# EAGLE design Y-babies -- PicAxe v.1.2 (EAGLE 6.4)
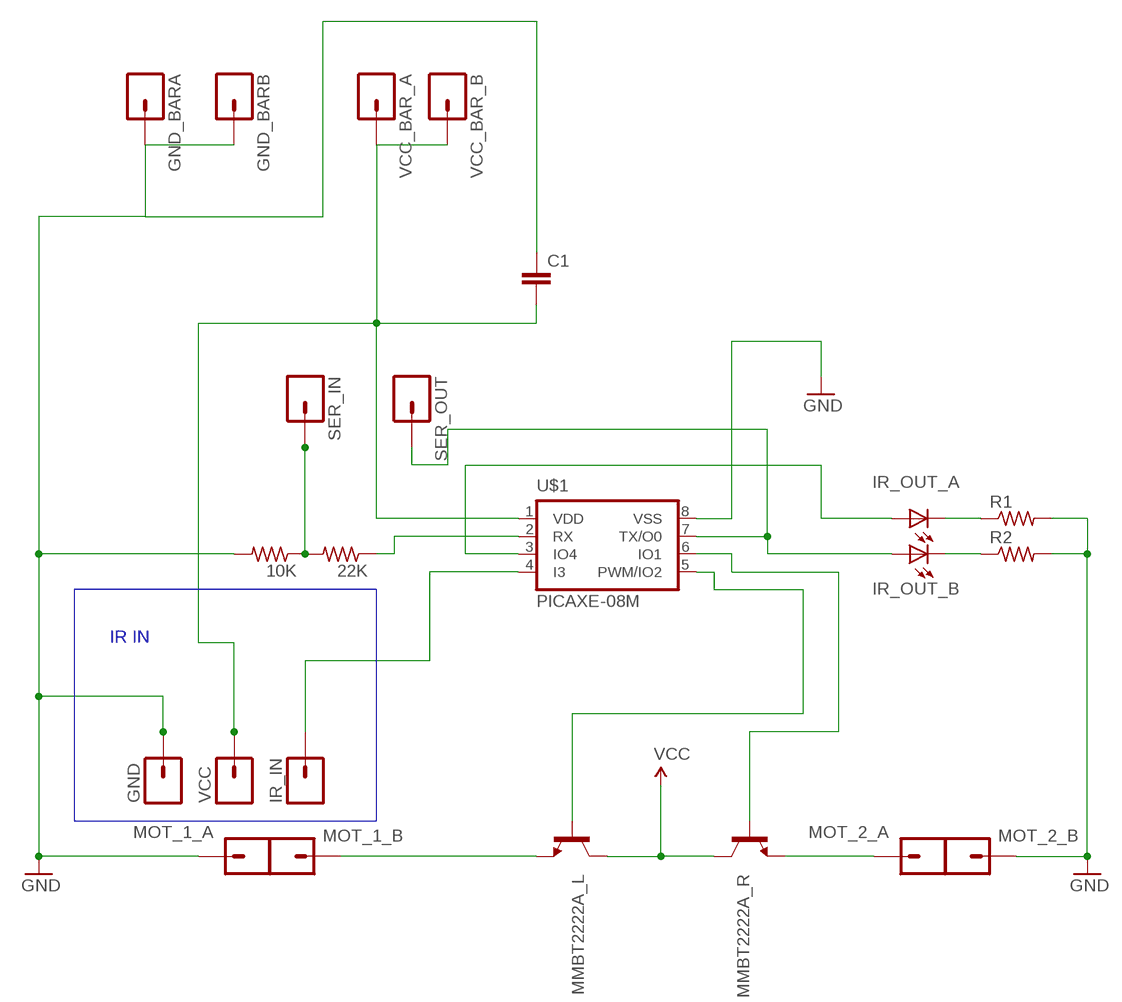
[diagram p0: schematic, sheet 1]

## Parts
10K  R-US_R0805W  [R0805W]
22K  R-US_R0805W  [R0805W]
C1  CAPPTH1  [CAP-PTH-5MM]
GND  M01PTH  [1X01]
GND_BARA  M01PTH  [1X01]
GND_BARB  M01PTH  [1X01]
IR_IN  M01PTH  [1X01]
IR_OUT_A  LED3MM  [LED3MM]
IR_OUT_B  LED3MM  [LED3MM]
MMBT2222A_L  TRANSISTOR_NPNSOT23  [SOT23]
MMBT2222A_R  TRANSISTOR_NPNSOT23  [SOT23]
MOT_1_A  M01SMD-4.5X1.5  [PAD-1.5X4.5]
MOT_1_B  M01SMD-4.5X1.5  [PAD-1.5X4.5]
MOT_2_A  M01SMD-4.5X1.5  [PAD-1.5X4.5]
MOT_2_B  M01SMD-4.5X1.5  [PAD-1.5X4.5]
R1  R-US_R0805W  [R0805W]
R2  R-US_R0805W  [R0805W]
SER_IN  M01PTH  [1X01]
SER_OUT  M01PTH  [1X01]
U$1  PICAXE-08M  [DIL8]
VCC  M01PTH  [1X01]
VCC_BAR_A  M01PTH  [1X01]
VCC_BAR_B  M01PTH  [1X01]

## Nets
GND: 10K.2 C1.1 GND.1 GND_BARA.1 GND_BARB.1 MOT_1_A.P$1 MOT_2_B.P$1 R1.2 R2.2 U$1.8(VSS)
N$1: MMBT2222A_L.1(B) U$1.5(PWM/IO2)
N$2: MMBT2222A_R.1(B) U$1.6(IO1)
N$3: IR_OUT_B.A SER_OUT.1 U$1.7(TX/O0)
N$4: IR_OUT_B.K(C) R2.1
N$5: 10K.1 22K.2 SER_IN.1
N$6: IR_OUT_A.A U$1.3(IO4)
N$7: IR_OUT_A.K(C) R1.1
N$8: 22K.1 U$1.2(RX)
N$9: MMBT2222A_L.2(E) MOT_1_B.P$1
N$10: MMBT2222A_R.2(E) MOT_2_A.P$1
N$11: IR_IN.1 U$1.4(I3)
VCC: C1.2 MMBT2222A_L.3(C) MMBT2222A_R.3(C) U$1.1(VDD) VCC.1 VCC_BAR_A.1 VCC_BAR_B.1

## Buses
B$1

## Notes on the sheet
- IR IN

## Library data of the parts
10K 22K R1 R2 = resistor:R-US_: RESISTOR, American symbol
C1 = SparkFun:CAP: Capacitor
GND GND_BARA GND_BARB IR_IN MOT_1_A MOT_1_B MOT_2_A MOT_2_B SER_IN SER_OUT VCC VCC_BAR_A VCC_BAR_B = SparkFun:M01: Header 1
IR_OUT_A IR_OUT_B = led:LED: LED
MMBT2222A_L MMBT2222A_R = SparkFun:TRANSISTOR_NPN: Transistor NPN BJT configuration in SOT23 package. MMBT2222 is the common NPN we use. Double check BCE configuration again layout.
U$1 = picaxe-3:PICAXE-08M

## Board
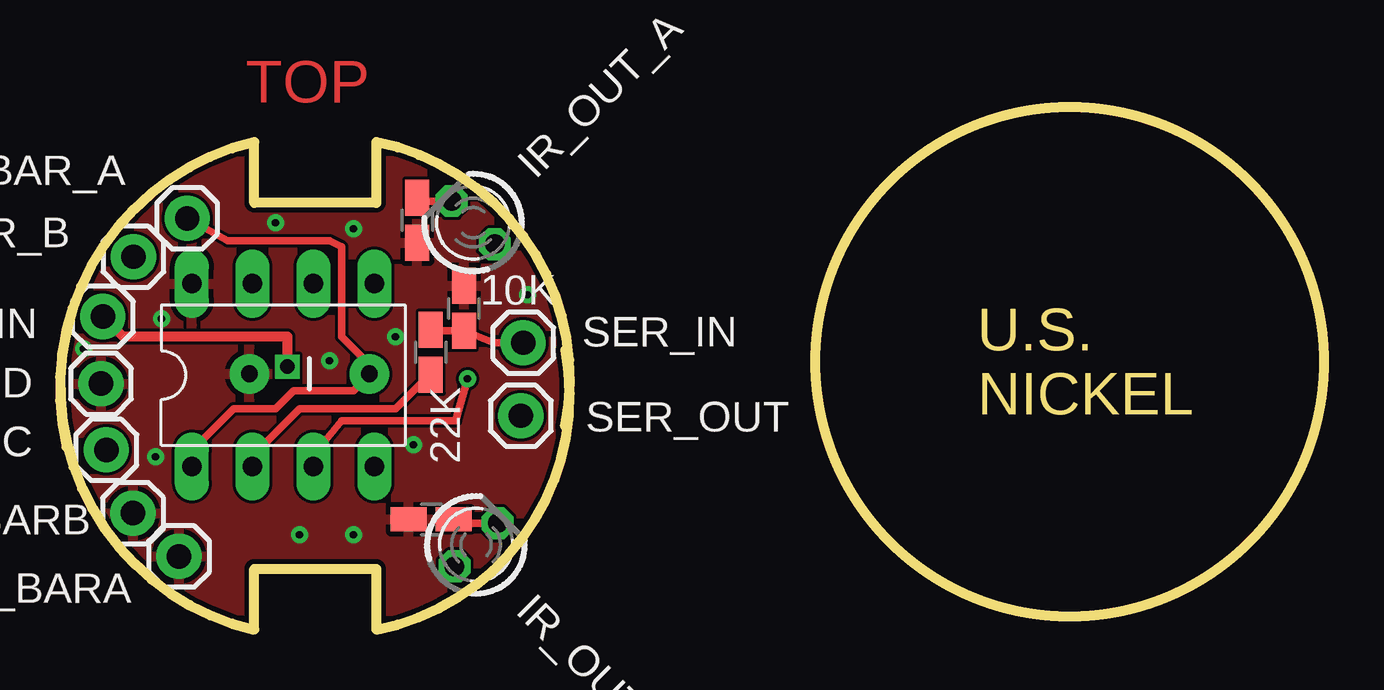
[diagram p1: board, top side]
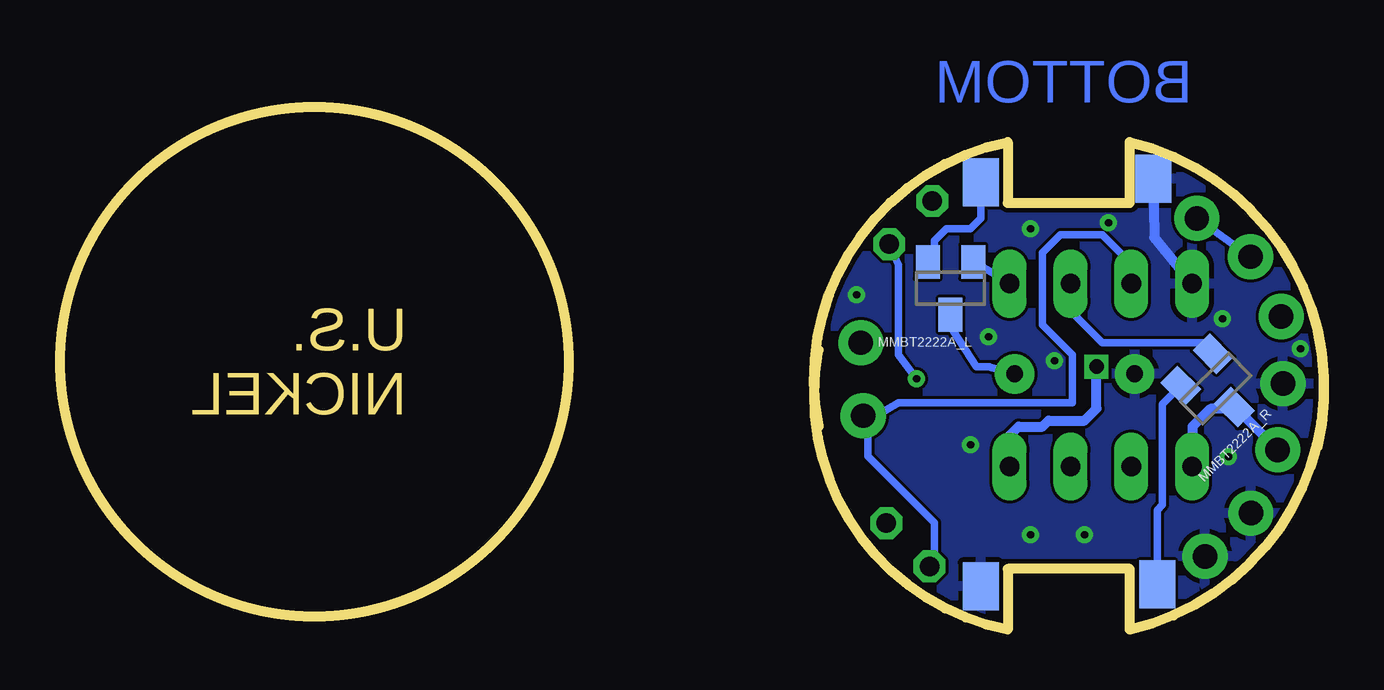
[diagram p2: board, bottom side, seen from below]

Size 52.69 x 21.77 mm. Coordinates in mm from the lower left corner, seen from the top.
Outline: 0.27,7.62 arc-90 8.1,20.32 8.1,17.78 13.18,17.78 13.18,20.32 arc-90 21.06,8.46
Outline: 0.27,12.48 arc90 8.1,0 8.1,2.54 13.18,2.54 13.18,0 arc90 21.07,11.66
Outline: circle at 42.08,11.16 radius 10.61
Copper layers (1*16): Top 0.035mm / dielectric 1.5mm / Bottom 0.035mm
Design rules "default *": minimum track width 10mil, minimum drill 24mil, track to track 5mil, track to pad 5mil, pad to pad 5mil, via to via 5mil, smd to smd 5mil, copper to edge 8mil, drill to drill 6mil, minimum pad ring 10mil, minimum via ring 8mil, stop-mask expansion 4mil, vias tented up to drill 0.3mm, thermal gap 8mil

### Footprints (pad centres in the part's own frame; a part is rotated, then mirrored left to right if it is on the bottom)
R0805W = smd 1.5 x 1: 1 -0.94,0; 2 0.94,0
CAP-PTH-5MM = drill 0.7 pad 1.651: 1 -2.5,0; 2 2.5,0
1X01 = drill 1.016 pad 1.88: 1 0,0
LED3MM = drill 0.813 octagon: A -1.27,0; K 1.27,0
SOT23 = smd 1 x 1.4: 1 -0.95,-1.1; 2 0.95,-1.1; 3 0,1.1
PAD-1.5X4.5 = smd 1.5 x 2: P$1 0,0
DIL8 = drill 0.813 pad 1.422 long: 1 -3.81,-3.81; 2 -1.27,-3.81; 3 1.27,-3.81; 4 3.81,-3.81; 5 3.81,3.81; 6 1.27,3.81; 7 -1.27,3.81; 8 -3.81,3.81

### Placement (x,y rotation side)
10K  16.84,13.39 90 top
22K  15.46,11.56 90 top
C1  10.39,10.66 0 top
GND  1.71,10.26 0 top
GND_BARA  4.96,3.05 0 top
GND_BARB  3.04,4.86 0 top
IR_IN  1.79,13.05 0 top
IR_OUT_A  17.22,16.96 135 top
IR_OUT_B  17.34,3.54 45 top
MMBT2222A_L  15.57,14.22 180 bottom
MMBT2222A_R  4.51,10.05 225 bottom
MOT_1_A  7.12,18.78 0 bottom
MOT_1_B  14.29,18.65 180 bottom
MOT_2_A  6.96,1.89 180 bottom
MOT_2_B  14.31,1.81 0 bottom
R1  14.89,17.06 270 top
R2  15.48,4.6 180 top
SER_IN  19.31,11.96 0 top
SER_OUT  19.21,8.92 0 top
U$1  9.3,10.61 0 top
VCC  1.93,7.49 0 top
VCC_BAR_A  5.3,17.14 0 top
VCC_BAR_B  3.06,15.54 0 top

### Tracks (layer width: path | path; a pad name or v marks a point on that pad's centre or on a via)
GND  (via drill 0.3)
  Bottom 0.406: MOT_1_A.P$1 7.08,16.35 U$1.8
  other vias: 9.98,3.96 0.98,11.71 14.73,7.71 12.23,16.71 19.48,13.96 4.23,12.96 13.98,12.21 11.23,11.21 8.98,16.96 12.23,3.96 3.98,7.21
  pour Bottom: -0.79,20.32 -0.79,0 22.07,0 22.07,20.32
  pour Top: -0.79,20.32 -0.79,0 22.07,0 22.07,20.32
N$1
  Bottom 0.305: MMBT2222A_L.1 13.71,14.81 U$1.5
N$2
  Bottom 0.305: U$1.6 10.57,13.3 9.23,11.96 5.08,11.96 MMBT2222A_R.1
N$3
  Bottom 0.305: U$1.7 8.03,15.26 9.23,16.46 10.98,16.46 11.73,15.71 11.73,12.71 10.48,11.46 10.48,9.46 17.73,9.46 19,8.71 | 19,8.71 SER_OUT.1 | 19,8.71 19,7.23 16.23,4.46 16.23,2.85 IR_OUT_B.A
N$4
  Top 0.305: IR_OUT_B.K 16.58,4.44 R2.1
N$5
  Top 0.305: SER_IN.1 18.08,11.95 10K.1 15.51,12.45 22K.2
N$6  (via drill 0.3)
  Top 0.305: U$1.3 10.57,7.3 11.73,8.71 16.48,8.71 v16.98,10.46
  Bottom 0.305: v16.98,10.46 17.73,11.46 17.73,15.2 IR_OUT_A.A
N$7
  Top 0.305: IR_OUT_A.K 15.03,17.86 R1.1
N$8
  Top 0.305: U$1.2 8.03,7.26 9.98,9.21 13.98,9.21 15.23,10.46 15.3,10.46 22K.1
N$9
  Bottom 0.305: MOT_1_B.P$1 14.29,17.15 14.73,16.71 15.73,16.71 16.23,16.21 16.23,15.61 MMBT2222A_L.2
N$10
  Bottom 0.305: MOT_2_A.P$1 6.96,4.99 6.73,5.21 6.73,9.39 MMBT2222A_R.2
N$11  (via drill 0.6)
  Top 0.406: v9.48,10.96 9.48,12.21 2.63,12.21 IR_IN.1
  Bottom 0.406: U$1.4 13.11,8.08 12.73,8.46 11.73,8.46 11.48,8.71 9.98,8.71 9.48,9.21 v9.48,10.96
VCC
  Top 0.305: 12.98,10.71 12.98,10.96 11.73,12.21 11.73,15.96 11.23,16.21 6.98,16.21 VCC_BAR_A.1 | 5.48,7.46 7.23,9.21 8.98,9.21 9.73,9.96 12.23,9.96 12.98,10.71 | 12.98,10.71 12.94,10.71 C1.2
  Top 0.406: U$1.1 5.49,7.45 5.48,7.46
  Bottom 0.305: MMBT2222A_L.3 15.45,12.43 14.48,10.96 13.98,10.96 | 13.98,10.96 13.94,10.96 | C1.2 12.93,10.66 13.98,10.96 | VCC_BAR_A.1 VCC_BAR_B.1 2.73,14.84 | MMBT2222A_R.3 3.74,9.2
  Bottom 0.406: VCC.1 3.64,9.2 3.74,9.2 4.74,9.2 5.48,8.46 U$1.1

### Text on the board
Top: TOP
Bottom: BOTTOM
Dimension: U.S. / NICKEL

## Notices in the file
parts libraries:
SparkFun: Licensing: CC v3.0 Share-Alike You are welcome to use this library for commercial purposes.
